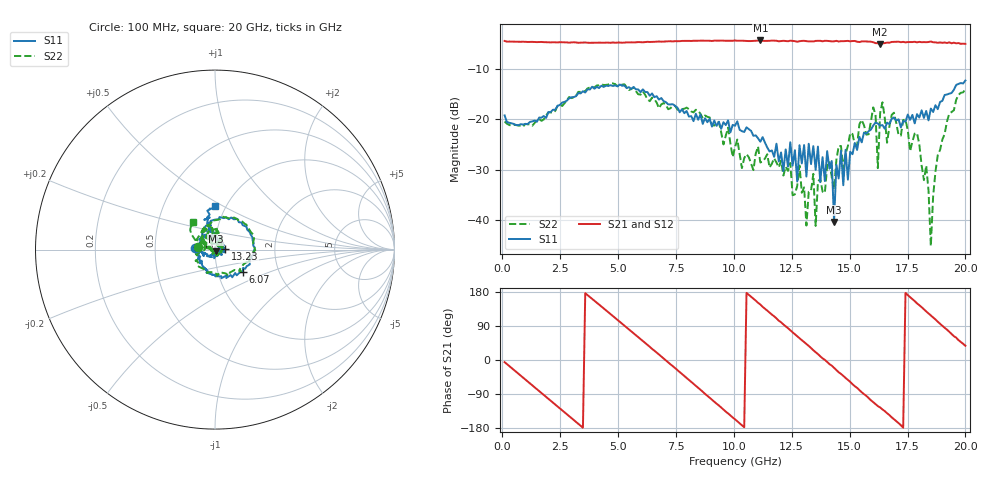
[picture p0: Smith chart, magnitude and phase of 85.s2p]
!Agilent Technologies,N5230C,MY49001569,A.09.33.09
!Agilent N5230C: A.09.33.09
!Date: Monday, July 27, 2015 14:18:46
!Correction: S11(Full 2 Port(1,2))
!S21(Full 2 Port(1,2))
!S12(Full 2 Port(1,2))
!S22(Full 2 Port(1,2))
!S2P File: Measurements: S11, S21, S12, S22:
# Hz S  dB  R 50
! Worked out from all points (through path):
!   201 points, 100 MHz to 20 GHz, reference 50 ohm
!   highest |S21| = -4.25 dB at 11.14 GHz (marker M1); lowest = -5.0 dB at 16.32 GHz (marker M2)
!   group delay of S21, straight-line fit = 145 ps
!   lowest |S11| = -40.4 dB at 14.33 GHz (marker M3), VSWR 1.02, Z = 50.4 - j0.884 ohm
!   |S11| at or under -10 dB: start of sweep to end of sweep
!   |S22| runs from -45.3 to -12.8 dB; largest |S21 - S12| = 0.019
!   S11 on the Smith chart (normalised r, x): 100 MHz: 0.80, +0.02; 6.07 GHz: 1.32, -0.34; 13.23 GHz: 1.12, +0.01; 20 GHz: 0.88, +0.46
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1e8  -19.19 174.8  -4.35 -5.7  -4.38 -5.7  -20.42 171.6
1.692e9  -19.64 134.5  -4.55 -87.3  -4.56 -87.4  -20.28 137.0
3.483e9  -14.38 71.0  -4.67 -178.5  -4.68 -178.9  -14.48 70.6
6.07e9  -14.00 -39.0  -4.62 50.0  -4.59 49.9  -14.41 -40.1
6.7665e9  -16.04 -65.3  -4.46 14.4  -4.48 14.0  -17.77 -76.9
8.5575e9  -19.04 -150.3  -4.29 -78.7  -4.29 -79.1  -18.84 -153.1
1.005e10  -21.26 144.7  -4.26 -156.4  -4.33 -157.3  -25.57 109.1
1.11445e10  -24.44 69.0  -4.25 146.3  -4.25 145.5  -28.59 45.7
1.3234e10  -24.85 2.5  -4.45 37.2  -4.41 36.2  -34.43 -120.6
1.3433e10  -25.33 -7.2  -4.45 25.9  -4.30 25.7  -30.85 -118.0
1.35325e10  -30.04 9.2  -4.34 20.5  -4.33 20.3  -41.23 158.5
1.4229e10  -28.29 -74.1  -4.43 -14.8  -4.43 -16.4  -31.55 172.5
1.43285e10  -40.44 -67.4  -4.43 -20.7  -4.43 -22.1  -33.89 158.8
1.4627e10  -26.24 -95.8  -4.39 -36.6  -4.38 -36.9  -25.29 156.3
1.602e10  -21.21 168.4  -4.60 -111.3  -4.63 -112.6  -17.59 121.0
1.6219e10  -20.82 172.4  -4.80 -121.8  -4.78 -122.4  -29.71 124.6
1.63185e10  -21.26 -177.7  -4.98 -125.2  -4.88 -126.9  -18.70 152.5
1.67165e10  -20.93 147.0  -4.70 -145.3  -4.60 -146.0  -21.41 127.6
1.79105e10  -18.94 101.6  -4.63 149.3  -4.61 149.4  -22.72 57.6
1.85075e10  -17.84 103.0  -4.46 117.5  -4.69 117.2  -45.27 31.6
1.8806e10  -17.95 105.2  -4.71 101.0  -4.63 100.9  -27.13 152.4
2e10  -12.24 90.6  -4.92 37.5  -5.01 37.0  -14.01 128.8
